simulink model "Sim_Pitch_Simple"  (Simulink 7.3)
settings: Solver=ode45  StartTime=0.0  StopTime=10  RelTol=1e-3
InitFcn:
  | init
StartFcn:
  | init
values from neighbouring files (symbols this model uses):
  r2d = 180/pi    (= 57.2957795131)    [init.m]    (also in robust.m)
undefined symbols (not defined in the file or in its folder): Aps, Bps, Cps, Dps, Kmix, Kq

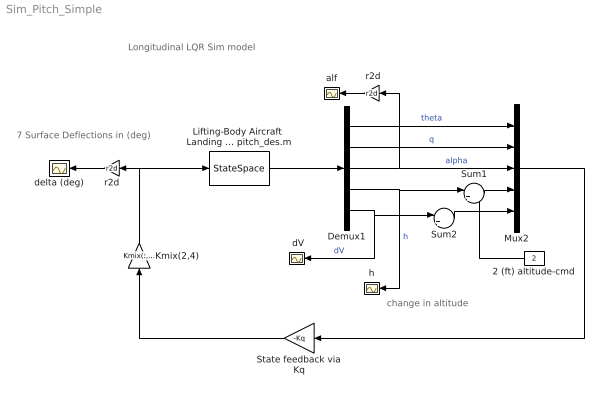
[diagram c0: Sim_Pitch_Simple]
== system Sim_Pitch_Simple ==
  note: Longitudinal LQR Sim model
  note: 7 Surface Deflections in (deg)
  note: change in altitude
  " dV" : Scope
  " r2d" : Gain  Gain=r2d  ParameterDataType=sfix(16)  ParameterScaling=2^0  OutDataType=sfix(16)  OutScaling=2^0
  2 (ft) altitude-cmd : Constant  Value=2  OutDataType=sfix(16)  OutScaling=2^0
  Demux1 : Demux  Outputs=5
  Kmix(2,4) : Gain  Gain=Kmix(:,[2,4])  Multiplication=Matrix(K*u)  ParameterDataType=sfix(16)  ParameterScaling=2^0  OutDataType=sfix(16)  OutScaling=2^0
  Lifting-Body Aircraft  Landing Phase  Pitch Design Model from file pitch_des.m : StateSpace  A=Aps  B=Bps  C=Cps  D=Dps
  Mux2 : Mux  Inputs=5
  State feedback via Kq : Gain  Gain=-Kq  Multiplication=Matrix(K*u)  ParameterDataType=sfix(16)  ParameterScaling=2^0  OutDataType=sfix(16)  OutScaling=2^0
  Sum1 : Sum  Inputs=|+-  OutDataType=sfix(16)  OutScaling=2^0
  Sum2 : Sum  Inputs=|+-  OutDataType=sfix(16)  OutScaling=2^0
  alf : Scope
  delta (deg) : Scope
  h : Scope
  r2d : Gain  Gain=r2d  ParameterDataType=sfix(16)  ParameterScaling=2^0  OutDataType=sfix(16)  OutScaling=2^0
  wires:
  Lifting-Body Aircraft  Landing Phase  Pitch Design Model from file pitch_des.m/1 -> Demux1/1
  Demux1/1 -> Mux2/1  "theta"
  Demux1/2 -> Mux2/2  "q"
  Mux2/1 -> State feedback via Kq/1
  State feedback via Kq/1 -> Kmix(2,4)/1
  Demux1/3 -> Mux2/3, " r2d"/1  "alpha"
  Sum1/1 -> Mux2/4
  Demux1/4 -> Sum1/1, h/1  "h"
  " r2d"/1 -> alf/1
  Sum2/1 -> Mux2/5
  Demux1/5 -> Sum2/1, " dV"/1  "dV"
  Kmix(2,4)/1 -> Lifting-Body Aircraft  Landing Phase  Pitch Design Model from file pitch_des.m/1, r2d/1
  r2d/1 -> delta (deg)/1
  2 (ft) altitude-cmd/1 -> Sum1/2
